FUNCTION_BLOCK Temp_controller
VAR_INPUT
	ENABLE:BOOL;
	AUTO_TUNE:BOOL;
	AUTO_TUNE_OUTPUT:REAL;
	//FILTER_ENABLE:BOOL;		
	TEMP_SV:REAL;
	TEMP_ACTUAL:REAL;
	
	TEMP_RATE:REAL;
	
	PID_P:REAL;
	PID_I:REAL;
	PID_D:REAL;
	PID_Dp:REAL;
	PID_Feedforward:REAL;
	PID_Output_Limit:REAL;
END_VAR
VAR_OUTPUT
	PID_AUTO_TUNE_P,
	PID_AUTO_TUNE_I,
	PID_AUTO_TUNE_D:REAL;
	PID_AUTO_TUNE_DONE:BOOL;
	SCR_OUT: REAL;
	SSR_ON:BOOL;
END_VAR
VAR
	SAMPLING_TIME:TIME:=T#1S;	//采样时间
	
	PID_NM : FB_CTRL_PID;
	PID_PARAMS:ST_CTRL_PID_PARAMS;
	PID_MODE:E_CTRL_MODE;
	PID_OUTPUT:LREAL;
	PID_FUC_STATE:E_CTRL_STATE;
	PID_ERRID:E_CTRL_ERRORCODES;
	PID_ERR:BOOL;
	PID_TASKTIME:TIME:=T#800MS;
	PID_CYCLETIME:TIME:=T#800MS;
	
	SSR_ON_PERCENT:REAL;
	
	TEMP_DATA_ARR : ARRAY[1..10] OF REAL;	//FIFO
	
	FIRST_RUN:R_TRIG;
	
	SAMPLING_TON1:TON;
	SAMPLING_TON2:TON;
	SAMPLING_TON1_EN:BOOL;
	SAMPLING_TON2_EN:BOOL;
	
	TEMP_AVERAGE:REAL;
	
	i: INT;
	
	SSR_ON_TIME:TIME;
	SSR_RESET_TIME:TIME;
	SSR_ON_TON:TON;
	SSR_RESET_TON:TON;
	SSR_ON_ENABLE:BOOL;
	SSR_RESET_ENABLE:BOOL;
	
	PID_AUTO_TUNE:PID_AutoTune;
	
	TON_FOR_RATE:TON;
	CACHE_TEMP_SV:REAL;
	TEMP_SV_TO_PID:REAL;
	EACH_STEP_TEMP:REAL;

END_VAR

//TEMP_RATE
EACH_STEP_TEMP:=TEMP_RATE/10;
IF TEMP_RATE=0 THEN 
	TEMP_SV_TO_PID:=TEMP_SV;
	ELSE
		IF ENABLE AND TON_FOR_RATE.IN=FALSE AND CACHE_TEMP_SV<TEMP_SV THEN
			TON_FOR_RATE.IN:=TRUE;
		END_IF			
		IF 	TON_FOR_RATE.Q THEN
			CACHE_TEMP_SV:=CACHE_TEMP_SV+EACH_STEP_TEMP;
			TON_FOR_RATE.IN:=FALSE;
		END_IF
			TON_FOR_RATE(IN:=, PT:= T#6S, Q=> , ET=> );
		IF CACHE_TEMP_SV<TEMP_SV THEN
			TEMP_SV_TO_PID:=CACHE_TEMP_SV;
		ELSE 
			TEMP_SV_TO_PID:=TEMP_SV;
		END_IF
END_IF

IF TEMP_RATE=0 OR NOT ENABLE THEN 
	CACHE_TEMP_SV:=0;
END_IF

IF (TEMP_RATE<>0) AND ENABLE AND (CACHE_TEMP_SV=0 OR CACHE_TEMP_SV>TEMP_SV) THEN 
	CACHE_TEMP_SV:=TEMP_AVERAGE+EACH_STEP_TEMP;
END_IF



//数组数据初始化
FIRST_RUN(CLK:=ENABLE,Q=> );
IF FIRST_RUN.Q
	THEN
	SAMPLING_TON1_EN:=TRUE;
	FOR i:=1  TO 10 BY 1
	DO
	TEMP_DATA_ARR[i] := TEMP_ACTUAL;
	END_FOR;
END_IF;

//产生采样脉冲
SAMPLING_TON1(IN:=SAMPLING_TON1_EN , PT:=SAMPLING_TIME , Q=> , ET=> );
IF SAMPLING_TON1.Q 
	THEN
	SAMPLING_TON1_EN:=0;
	SAMPLING_TON2_EN:=1;
END_IF;
SAMPLING_TON2(IN:=SAMPLING_TON2_EN , PT:=SAMPLING_TIME , Q=> , ET=> );
IF SAMPLING_TON2.Q 
	THEN 
	SAMPLING_TON1_EN:=1;
	SAMPLING_TON2_EN:=0;
END_IF;

//数组右移一位
IF SAMPLING_TON1.Q OR SAMPLING_TON2.Q		
	THEN 
	TEMP_DATA_ARR[10]	:= 	TEMP_DATA_ARR[9];
	TEMP_DATA_ARR[9] 	:= 	TEMP_DATA_ARR[8];
	TEMP_DATA_ARR[8]	:= 	TEMP_DATA_ARR[7];
	TEMP_DATA_ARR[7] 	:= 	TEMP_DATA_ARR[6];
	TEMP_DATA_ARR[6] 	:=	TEMP_DATA_ARR[5];
	TEMP_DATA_ARR[5] 	:= 	TEMP_DATA_ARR[4];
	TEMP_DATA_ARR[4] 	:= 	TEMP_DATA_ARR[3];
	TEMP_DATA_ARR[3] 	:= 	TEMP_DATA_ARR[2];
	TEMP_DATA_ARR[2] 	:= 	TEMP_DATA_ARR[1];
	TEMP_DATA_ARR[1] 	:= 	TEMP_ACTUAL;
END_IF

//取平均数，前两个数据权重为0.5，中间4位权重为0.3，最后4位权重为0.2。原则上，时间越久，权重越小
	TEMP_AVERAGE:=0.5*(TEMP_DATA_ARR[1]+TEMP_DATA_ARR[2])/2
				 +0.3*(TEMP_DATA_ARR[3]+TEMP_DATA_ARR[4]+TEMP_DATA_ARR[5]+TEMP_DATA_ARR[6])/4
				 +0.2*(TEMP_DATA_ARR[7]+TEMP_DATA_ARR[8]+TEMP_DATA_ARR[9]+TEMP_DATA_ARR[10])/4;

	IF 	AUTO_TUNE
		THEN			 
			PID_MODE:=0;
		ELSE
			PID_MODE:=2;
	END_IF;

	PID_AUTO_TUNE(
		PV:= TEMP_ACTUAL, 
		AutoTuneActive:= AUTO_TUNE, 
		StepResponseAmplitude:=AUTO_TUNE_OUTPUT,
		Output=> 	, 
		Kp=> 		PID_AUTO_TUNE_P, 
		Ki=> 		PID_AUTO_TUNE_I, 
		Kd=> 		PID_AUTO_TUNE_D, 
		Done=> 		PID_AUTO_TUNE_DONE);
		
//*******PID的背景数据块							G(S)=Kp[1+1/Tn+Tv/(1+Td)]
	PID_PARAMS.tTaskCycleTime		:=T#10MS;			//任务周期
	PID_PARAMS.tCtrlCycleTime		:=T#500MS;			//控制循环时间
	PID_PARAMS.fKp					:=PID_P;			//P
	PID_PARAMS.tTn					:=REAL_TO_TIME(PID_I*1000);			//I
	PID_PARAMS.tTv					:=REAL_TO_TIME(PID_D*1000);			//D
	PID_PARAMS.tTd					:=REAL_TO_TIME(PID_Dp*1000);			//DAMP阻尼时间
	PID_PARAMS.fOutMaxLimit			:=100;				//输出上限
	PID_PARAMS.fOutMinLimit			:=0;				//输出下限
	PID_PARAMS.bPInTheFeedbackPath	:=FALSE;			//P有效
	PID_PARAMS.bDInTheFeedbackPath	:=FALSE;			//D有效
	PID_PARAMS.bARWOnIPartOnly		:=FALSE;			//I有效

//PID函数
	PID_NM(
		fSetpointValue:= TEMP_SV_TO_PID, 						//设定值
		fActualValue:= TEMP_ACTUAL, 					//实际值
		fManSyncValue:= , 								//操作值
		bSync:= , 										//上升沿时，操作值有效
		eMode:= PID_MODE, 								//函数的运行模式，0:空闲,1:PASSIVE,2:ACTIVE,3:RESET,4:MANUAL,5:AUTO,6:SELF-TUNING,7:SYNC同步模式
		bHold:= , 										//TRUE时，保持当前的内部状态
		fOut=> PID_OUTPUT, 								//输出值
		bARWactive=> , 									//TRUE时，表示PID输出值被限制
		eState=> PID_FUC_STATE, 						//函数状态
		eErrorId=> PID_ERRID, 							//ERR代码
		bError=> PID_ERR, 								//PID发生错误
		stParams:=PID_PARAMS );
		
	IF AUTO_TUNE 
		THEN 
		SSR_ON_PERCENT:=PID_AUTO_TUNE.Output+PID_Feedforward;		
		ELSE
		SSR_ON_PERCENT:=LREAL_TO_REAL(PID_OUTPUT+PID_Feedforward);
	END_IF
	
	IF SSR_ON_PERCENT>PID_Output_Limit AND ENABLE
		THEN 
		SSR_ON_PERCENT:=PID_Output_Limit;
	END_IF	
	IF SSR_ON_PERCENT<0 OR NOT ENABLE
		THEN 
		SSR_ON_PERCENT:=0;
	END_IF	

	SCR_OUT:=SSR_ON_PERCENT;
	
//*******PWM脉冲输出生成	
	
	SSR_ON_TIME:=REAL_TO_TIME(SSR_ON_PERCENT*10);									//输出脉冲ON宽度
	SSR_RESET_TIME:=REAL_TO_TIME((100-SSR_ON_PERCENT)*10);							//输出脉冲总宽度
	SSR_ON_TON(IN:= SSR_ON_ENABLE, PT:= SSR_ON_TIME, Q=> , ET=> );					//输出脉冲计时
	IF SSR_ON_TON.Q 																//输出脉冲计时器使能在计时器下方ON，实现上升脉冲；同时复位计时器使能OFF
		THEN 
		SSR_RESET_ENABLE:=TRUE;
	END_IF
	IF NOT (SSR_ON_ENABLE OR SSR_RESET_ENABLE)										//首次cycle触发输出脉冲使能
		THEN
		SSR_ON_ENABLE:=TRUE;
	END_IF
	SSR_RESET_TON(IN:= SSR_RESET_ENABLE, PT:= SSR_RESET_TIME, Q=> , ET=> );
	IF SSR_RESET_TON.Q 
		THEN 
		SSR_ON_ENABLE:=FALSE;
		SSR_RESET_ENABLE:=FALSE;
		SSR_ON:=FALSE;																//输出脉冲计时器使能OFF
	END_IF
	IF SSR_ON_PERCENT>0
		THEN 
		SSR_ON:=NOT SSR_ON_TON.Q;
	END_IF

END_FUNCTION_BLOCK
